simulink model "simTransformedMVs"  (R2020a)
settings: Solver=VariableStepAuto  StartTime=0.0  StopTime=tsim  RelTol=1e-3
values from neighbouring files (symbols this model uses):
  KcT = 1/kT*tauT/(taucT)    [runTransformedMVs.m]
  KIq = 1/(taucq)    (= 0.5)    [runTransformedMVs.m]
  OL = 1    [SetUpSimulations.m]
  p = [V;A;B; transf]    [runTransformedMVs.m]    (also in runTransformedMVsCascade.m; Main.m = [N, Fc0, rhoc, rhoh,U,A,cpc,cph]; Main_OL.m = [N, Fc0, rhoc, rhoh,U,A,cpc,cph]; runTestCalcBlk.m = [N, Fc0, rhoc, rhoh,U,A,cpc,cph])
  q0 = 10    [SetUpSimulations.m]
  qstep = q0 + 2    (= 12)    [SetUpSimulations.m]
  T0 = 35    [SetUpSimulations.m]    (also in H2P_Turbine_driven.m = param(9); runTD.m = 318; H2P_Boiler_driven.m = param(9); runBD.m = 318)
  T10 = 20    [SetUpSimulations.m]
  T1m = T10    (= 20)    [SetUpSimulations.m]
  T1step = T10 + 10    (= 30)    [SetUpSimulations.m]
  T20 = 50    [SetUpSimulations.m]
  T2m = T20    (= 50)    [SetUpSimulations.m]
  T2step = T20 + 10    (= 60)    [SetUpSimulations.m]
  tauIT = min(-1/A, 4*(taucT))    [runTransformedMVs.m]
  Tstep = T0 + 10    (= 45)    [SetUpSimulations.m]
  tstep_q = 50    [SetUpSimulations.m]
  tstep_T = 100    [SetUpSimulations.m]
  tstep_T1 = 150    [SetUpSimulations.m]
  tstep_T2 = 200    [SetUpSimulations.m]
  vqbias = q0    [runTransformedMVs.m]    (also in runTransformedMVsCascade.m)
  vqbias_step = vqbias    [runTransformedMVs.m]    (also in runTransformedMVsCascade.m)
  vTbias = -A/B*T0    [runTransformedMVs.m]    (also in runTransformedMVsCascade.m)
  vTbias_step = vTbias    [runTransformedMVs.m]    (also in runTransformedMVsCascade.m)
undefined symbols (not defined in the file or in its folder): InputTransf, InvInputTransf, TempMixDAE

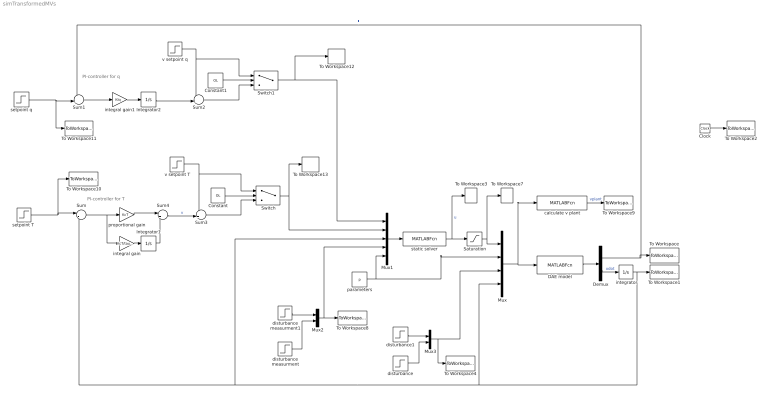
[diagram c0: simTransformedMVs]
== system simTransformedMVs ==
  note: PI-controller for T
  note: PI-controller for q
  " integrator" : Integrator  InitialCondition=T0
  Clock : Clock
  Constant : Constant  Value=OL
  Constant1 : Constant  Value=OL
  DAE model : MATLABFcn  MATLABFcn=TempMixDAE(u(1:2), u(3:6),u(7:8),u(9))  OutputDimensions=2
  Demux : Demux  Outputs=2
  Integrator1 : Integrator
  Integrator2 : Integrator
  Mux : Mux
  Mux1 : Mux  Inputs=5
  Mux2 : Mux  Inputs=2
  Mux3 : Mux  Inputs=2
  Saturation : Saturate  UpperLimit=inf  LowerLimit=-inf
  Sum : Sum  Inputs=|+-
  Sum1 : Sum  Inputs=-+|
  Sum2 : Sum  Inputs=++|
  Sum3 : Sum  Inputs=++|
  Sum4 : Sum  Inputs=|++
  Switch : Switch  Criteria=u2 > Threshold
  Switch1 : Switch  Criteria=u2 > Threshold
  To Workspace : ToWorkspace  VariableName=q  SampleTime=-1
  To Workspace1 : ToWorkspace  VariableName=T  SampleTime=-1
  To Workspace10 : ToWorkspace  VariableName=Tsp  SampleTime=-1
  To Workspace11 : ToWorkspace  VariableName=qsp  SampleTime=-1
  To Workspace12 : ToWorkspace  VariableName=vqs  SampleTime=-1
  To Workspace13 : ToWorkspace  VariableName=vTs  SampleTime=-1
  To Workspace2 : ToWorkspace  VariableName=time  SampleTime=-1
  To Workspace3 : ToWorkspace  VariableName=u  SampleTime=-1
  To Workspace4 : ToWorkspace  VariableName=d  SampleTime=-1
  To Workspace7 : ToWorkspace  VariableName=uplant  SampleTime=-1
  To Workspace8 : ToWorkspace  VariableName=dm  SampleTime=-1
  To Workspace9 : ToWorkspace  VariableName=v  SampleTime=-1
  calculate v plant : MATLABFcn  MATLABFcn=InputTransf(u(1:2),u(3:6),u(7:8),u(9))  OutputDimensions=2
  disturbance : Step  Time=tstep_T2  Before=T20  After=T2step  SampleTime=0
  disturbance measurment : Step  Time=tstep_T2  Before=T20  After=T2m  SampleTime=0
  disturbance measurment1 : Step  Time=tstep_T1  Before=T10  After=T1m  SampleTime=0
  disturbance1 : Step  Time=tstep_T1  Before=T10  After=T1step  SampleTime=0
  integral gain : Gain  Gain=KcT/tauIT  Multiplication=Matrix(K*u)
  integral gain1 : Gain  Gain=KIq  Multiplication=Matrix(K*u)
  parameters : Constant  Value=p
  proportional gain : Gain  Gain=KcT  Multiplication=Matrix(K*u)
  "setpoint T " : Step  Time=tstep_T  Before=T0  After=Tstep  SampleTime=0
  setpoint q : Step  Time=tstep_q  Before=q0  After=qstep  SampleTime=0
  static solver : MATLABFcn  MATLABFcn=InvInputTransf(u(1:2),u(3),u(4:5),u(6:9))  OutputDimensions=2
  v setpoint T : Step  Time=tstep_T  Before=vTbias  After=vTbias_step  SampleTime=0
  v setpoint q : Step  Time=tstep_q  Before=vqbias  After=vqbias_step  SampleTime=0
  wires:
  DAE model/1 -> Demux/1
  Demux/1 -> To Workspace/1, Sum1/1  "F"
  " integrator"/1 -> To Workspace1/1, Mux/4, Sum/2, Mux1/3  "T"
  Mux/1 -> calculate v plant/1, DAE model/1
  Clock/1 -> To Workspace2/1
  Mux1/1 -> static solver/1
  Demux/2 -> " integrator"/1  "xdot"
  parameters/1 -> Mux/2, Mux1/5
  disturbance/1 -> Mux3/2
  static solver/1 -> Saturation/1, To Workspace3/1  "u"
  Saturation/1 -> To Workspace7/1, Mux/1
  Mux2/1 -> To Workspace8/1, Mux1/4
  calculate v plant/1 -> To Workspace9/1  "vplant"
  disturbance measurment1/1 -> Mux2/1
  disturbance measurment/1 -> Mux2/2
  disturbance1/1 -> Mux3/1
  Mux3/1 -> To Workspace4/1, Mux/3
  Sum4/1 -> Sum3/2  "v"
  v setpoint T/1 -> Sum3/1, Switch/1
  "setpoint T "/1 -> Sum/1, To Workspace10/1
  proportional gain/1 -> Sum4/1
  integral gain/1 -> Integrator1/1
  Sum/1 -> integral gain/1, proportional gain/1
  Integrator1/1 -> Sum4/2
  Switch/1 -> To Workspace13/1, Mux1/2
  Sum3/1 -> Switch/3
  Constant/1 -> Switch/2
  Constant1/1 -> Switch1/2
  setpoint q/1 -> Sum1/2, To Workspace11/1
  Sum2/1 -> Switch1/3
  integral gain1/1 -> Integrator2/1
  Integrator2/1 -> Sum2/2
  Sum1/1 -> integral gain1/1
  v setpoint q/1 -> Sum2/1, Switch1/1
  Switch1/1 -> To Workspace12/1, Mux1/1
